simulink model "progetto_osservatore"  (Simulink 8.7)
settings: Solver=VariableStepAuto  SolverMode=SingleTasking  StartTime=0.0  StopTime=10  RelTol=1e-3
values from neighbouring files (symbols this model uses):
  A = [0.9944 -0.1203 -0.4302    [esempio_progetto_oss_SISO.m]
  Ao = A - K*C    [esempio_progetto_oss_SISO.m]
  B = [0.4252 -0.0082 0.1813]'    [esempio_progetto_oss_SISO.m]
  Bo = [B K]    [esempio_progetto_oss_SISO.m]
  C = [1 0 0]    [esempio_progetto_oss_SISO.m]
  Co = C    [esempio_progetto_oss_SISO.m]
  D = zeros(m,r)    [esempio_progetto_oss_SISO.m]
  Do = zeros(m,r+m)    [esempio_progetto_oss_SISO.m]
  Tc = 0.1    [esempio_progetto_oss_SISO.m]
  x0 = 0.05    [esempio_progetto_oss_SISO.m]

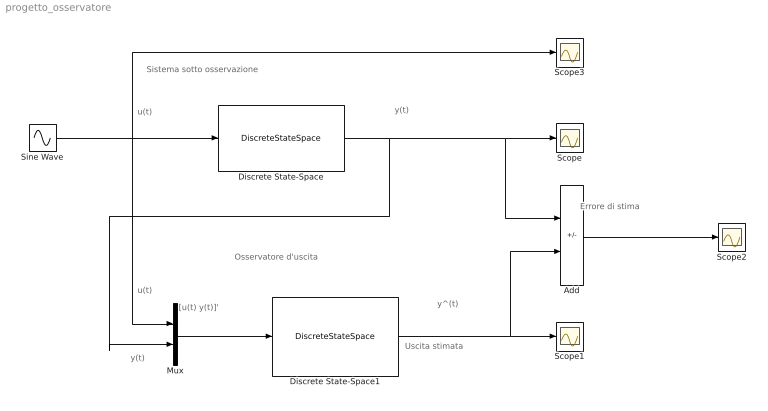
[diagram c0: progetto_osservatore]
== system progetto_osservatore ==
  note: Errore di stima
  note: y^(t)
  note: Uscita stimata
  note: [u(t) y(t)]'
  note: y(t)
  note: u(t)
  note: Osservatore d'uscita
  note: Sistema sotto osservazione
  note: y(t)
  note: u(t)
  Add : Sum  Inputs=+-
  Discrete State-Space : DiscreteStateSpace  A=A  B=B  C=C  D=D  X0=x0  SampleTime=Tc
  Discrete State-Space1 : DiscreteStateSpace  A=Ao  B=Bo  C=Co  D=Do  SampleTime=Tc
  Mux : Mux  Inputs=2
  Scope{,1..3} (4 alike) : Scope
  Sine Wave : Sin  SampleTime=0
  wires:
  Sine Wave/1 -> Scope3/1, Mux/1, Discrete State-Space/1
  Discrete State-Space/1 -> Mux/2, Add/1, Scope/1
  Mux/1 -> Discrete State-Space1/1
  Discrete State-Space1/1 -> Add/2, Scope1/1
  Add/1 -> Scope2/1
